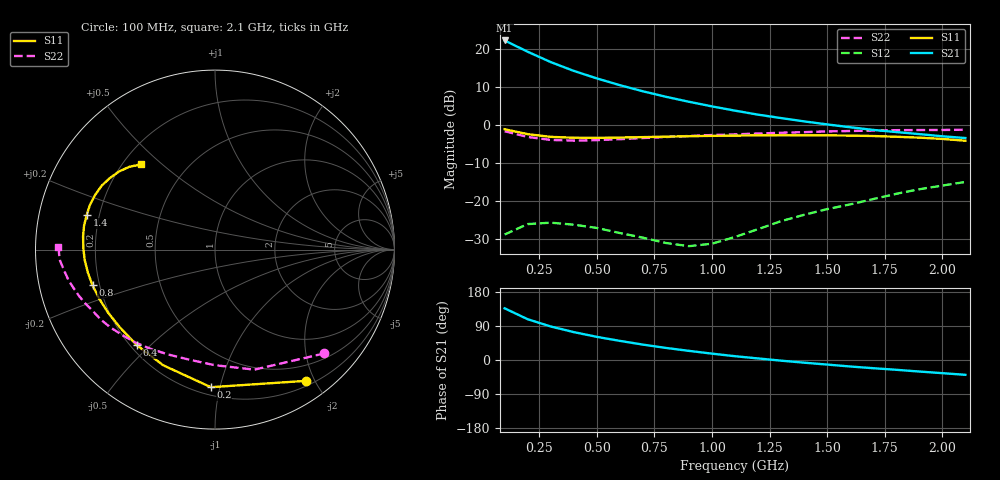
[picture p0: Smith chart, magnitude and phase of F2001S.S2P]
! Date: Fri Aug 11 12:06:03 1995
# MHZ  S  MA  R  50.0000
!  POLYFET RF DEVICES
!  F2001S
!  S PARAMETERS
!  VDS=28V, IDQ=800mA
! FREQ  S11MAG  S11ANG  S21MAG  S21ANG  S12MAG  S12ANG  S22MAG  S22ANG
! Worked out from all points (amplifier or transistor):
!   21 points, 100 MHz to 2.1 GHz, reference 50 ohm
!   highest |S21| = 22.4 dB at 100 MHz (marker M1)
!   |S21| within 3 dB of that: start of sweep to 201.1 MHz
!   unconditionally stable (mu >= 1): 665.4 MHz to 1.238 GHz
!   at 400 MHz: K = 0.47, MSG = 20.3 dB, |S12| = -26.2 dB
!   at 1.1 GHz: K = 1.39, MAG = 12.9 dB, |S12| = -29.4 dB
!   at 2.1 GHz: K = 0.24, MSG = 5.8 dB, |S12| = -14.9 dB
!   S11 on the Smith chart (normalised r, x): 100 MHz: 0.27, -1.88; 200 MHz: 0.25, -0.94; 400 MHz: 0.22, -0.45; 800 MHz: 0.17, -0.14; 1.4 GHz: 0.15, +0.13; 2.1 GHz: 0.27, +0.43
100  0.8905 -55.2  13.15 136.4  0.03654 49.9  0.8394 -43.6
200  0.7669 -91.7  9.34 107.6  0.05013 26.6  0.7039 -71.8
300  0.7062 -114.2  6.824 88.5  0.05234 11.4  0.6439 -90.2
400  0.6879 -129.3  5.225 73.6  0.04922 3.3  0.6298 -103.4
500  0.6845 -140.5  4.162 61.1  0.04463 -2.7  0.6398 -114.0
600  0.6916 -149.5  3.389 50.5  0.03823 -3.5  0.6585 -122.8
700  0.7008 -157.0  2.815 40.7  0.03322 -0.3  0.682 -130.6
800  0.7109 -163.8  2.382 31.9  0.02826 9.2  0.7027 -137.4
900  0.7201 -169.8  2.048 24.1  0.02566 21.8  0.7253 -143.1
1000  0.7284 -175.4  1.779 16.8  0.02765 39.4  0.7464 -148.5
1100  0.7337 179.3  1.564 10.0  0.0339 50.1  0.762 -153.4
1200  0.7388 174.2  1.385 4.1  0.043 58.1  0.7812 -157.2
1300  0.7419 169.4  1.249 -1.7  0.05479 60.6  0.8002 -161.1
1400  0.7403 164.8  1.13 -7.1  0.06643 60.2  0.8154 -164.6
1500  0.7399 160.2  1.03 -12.0  0.07895 57.3  0.833 -168.0
1600  0.7338 155.4  0.945 -17.1  0.09109 55.1  0.8439 -170.9
1700  0.7246 150.5  0.872 -21.7  0.1071 53.0  0.8545 -173.6
1800  0.7087 145.9  0.817 -25.8  0.1256 49.5  0.8655 -175.9
1900  0.6899 141.0  0.7677 -30.4  0.1442 44.0  0.8689 -178.4
2000  0.6637 136.0  0.7188 -34.7  0.1611 39.2  0.8705 -179.9
2100  0.6279 130.9  0.6817 -39.1  0.1801 33.3  0.8774 178.9
